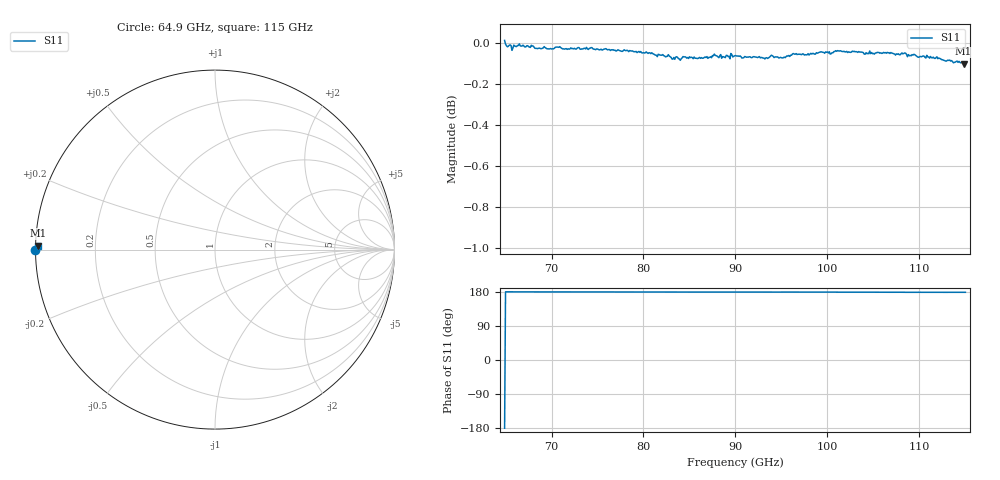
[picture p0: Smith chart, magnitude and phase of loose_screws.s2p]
# GHz S MA R 50
!freq magS11 angS11
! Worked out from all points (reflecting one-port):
!   502 points, 64.9 GHz to 115 GHz, reference 50 ohm
!   lowest |S11| = -0.1 dB at 114.8 GHz (marker M1), VSWR 169.36, Z = 0.295 + j0.574 ohm
!   phase of S11 starts at -180 deg and turns -1 deg over the sweep
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64.9  1.001 -180.0
65.4  0.9985 179.8
65.9  0.9986 179.8
66.5  0.9992 179.9
68.4  0.9967 179.7
71.2  0.9964 179.6
77.5  0.9953 179.3
79.6  0.9945 179.2
83.7  0.9917 179.1
87.4  0.9915 179.4
88.5  0.9912 179.2
90  0.9928 179.3
90.7  0.9914 179.2
92  0.9921 179.2
93.2  0.9908 179.1
93.9  0.9929 179.2
95.2  0.9915 179.3
96.3  0.9939 179.3
99.9  0.9945 179.2
101.5  0.9952 178.9
102.5  0.9945 178.9
103.3  0.9945 179.0
106.2  0.9942 178.8
108.8  0.9933 178.7
110.1  0.9923 178.8
113.3  0.9902 178.6
114.8  0.9883 178.7
115  0.9889 178.7
